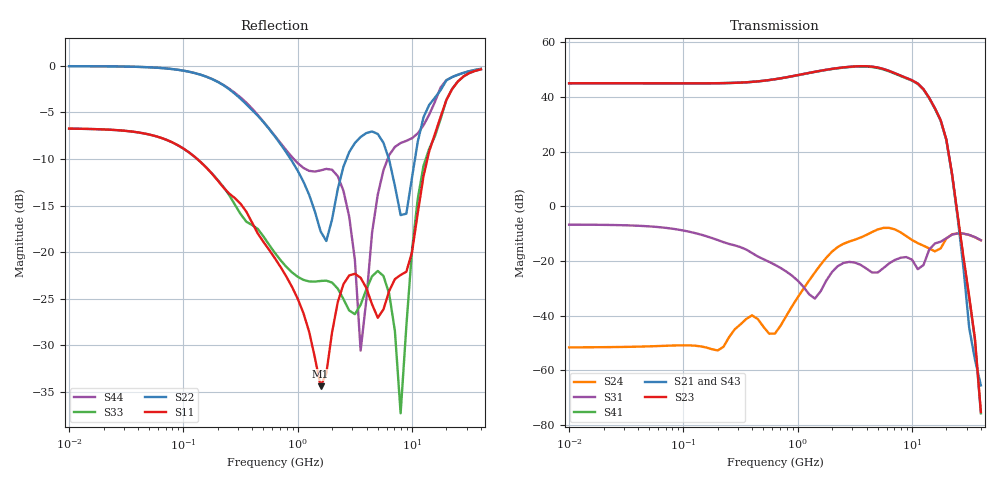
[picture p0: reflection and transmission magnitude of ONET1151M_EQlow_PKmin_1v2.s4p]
! Touchstone Ver. 1.0
! Thu Sep  6 15:44:44 2012
! Number of ports is 4
# Hz	S	DB	R	50.000000
! SCATTERING PARAMETERS  :
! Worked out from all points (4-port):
!   73 points, 10 MHz to 40 GHz, reference 50 ohm
!   strongest paths, dB at 10 MHz, 79.43 MHz, 631 MHz, 5.012 GHz, 40 GHz:
!     S23: 45.0, 45.0, 46.5, 50.8, -75.2
!     S21: 45.0, 45.0, 46.5, 50.8, -65.5
!     S43: 45.0, 45.0, 46.5, 50.6, -65.6
!     S41: 45.0, 45.0, 46.5, 50.6, -75.7
!     S31: -6.7, -8.1, -21.3, -24.2, -12.4
!     S24: -51.6, -50.9, -46.5, -8.4, -12.4
!   lowest |S11| = -34.4 dB at 1.585 GHz (marker M1), VSWR 1.04, Z = 51.2 - j1.52 ohm
!   |S11| at or under -10 dB: 132 MHz to 13.66 GHz (13.52 GHz wide, 196 % of centre)
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1e7  -6.75 -4.6  -110.76 178.2  -6.68 -4.3  -110.73 178.2
     45.02 -175.6  -0.04 7.1  45.02 4.4  -51.56 9.7
     -6.67 -4.3  -110.75 178.2  -6.75 -4.6  -110.75 178.2
     45.01 4.5  -51.49 9.8  45.01 -175.5  -0.04 7.1
1.584893e9  -34.39 -51.2  -40.82 67.1  -25.24 -56.1  -40.75 67.1
            49.60 132.9  -17.78 -78.2  49.60 -47.1  -21.33 78.4
            -31.05 15.9  -40.78 67.2  -23.10 -77.2  -40.75 67.1
            49.53 -47.6  -23.84 -80.6  49.53 132.4  -11.23 -85.8
3.981072e9  -23.85 -111.5  -38.52 -9.4  -23.76 44.2  -38.46 -9.2
            51.25 13.0  -7.22 -120.8  51.25 -167.0  -10.45 -128.3
            -22.72 -92.5  -38.51 -9.0  -23.98 66.0  -38.47 -9.3
            51.11 -167.7  -19.38 55.9  51.11 12.3  -25.14 -64.5
5.623413e9  -26.14 104.7  -37.92 -30.1  -29.08 -26.2  -37.87 -29.7
            50.25 -67.8  -8.27 168.9  50.24 112.3  -7.87 143.5
            -22.54 135.8  -37.90 -29.5  -22.57 -16.2  -37.85 -29.9
            50.06 111.7  -19.38 -132.3  50.05 -68.2  -11.20 -117.5
7.943282e9  -22.45 21.3  -38.41 -61.5  -22.34 97.8  -38.38 -61.0
            47.83 -172.4  -16.03 117.4  47.81 7.7  -9.48 67.3
            -18.77 67.0  -38.40 -60.9  -37.30 -15.2  -38.31 -61.6
            47.66 7.3  -8.95 114.9  47.64 -172.6  -8.29 155.7
1.122018e10  -15.81 25.8  -40.20 -97.7  -19.09 50.4  -40.21 -96.5
             44.92 38.2  -8.14 90.2  44.91 -141.5  -13.43 32.4
             -22.97 37.6  -40.29 -96.0  -14.26 35.7  -40.16 -98.0
             44.78 -142.2  -9.01 21.1  44.75 38.1  -7.25 68.9
4e10  -0.38 -143.6  -68.79 138.9  -12.36 -52.9  -68.60 138.8
      -65.45 -129.2  -0.33 -143.9  -75.20 -61.2  -12.41 -53.2
      -12.36 -52.9  -68.52 138.4  -0.38 -143.5  -68.78 139.1
      -75.66 -68.4  -12.40 -53.3  -65.61 -128.7  -0.33 -143.9
